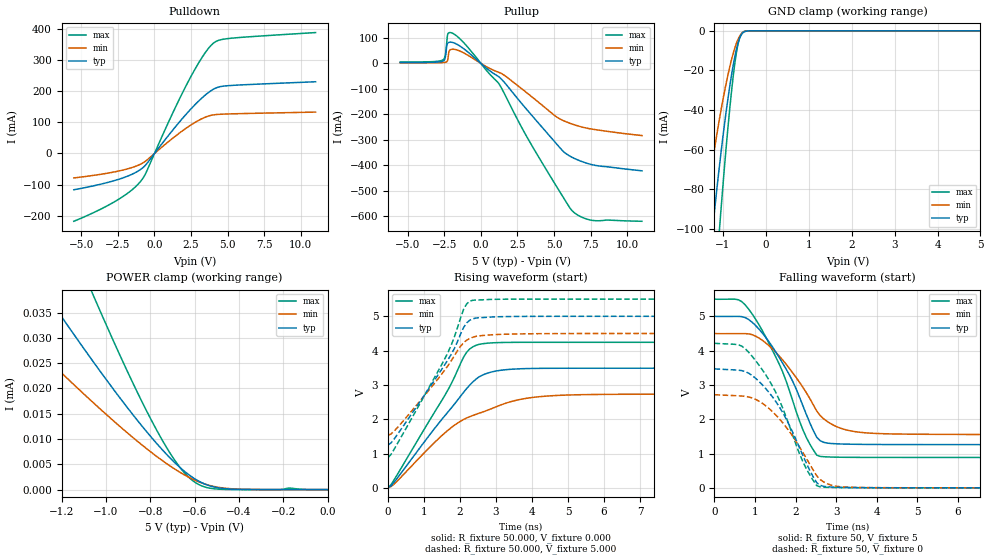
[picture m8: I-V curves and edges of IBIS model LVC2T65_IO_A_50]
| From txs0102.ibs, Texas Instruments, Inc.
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[Model]   LVC2T65_IO_A_50
Model_type  I/O
Vinl=0.15
Vinh=5.1
Enable   Active-High
Vref =   5
Rref =   1000000
Cref =   15p
Vmeas =   2.5
| variable   typ   min   max
C_comp   4.98pF   4.34pF   5.61pF
| C_pullup   5.82pF   4.29pF   6.44pF
| C_pulldown   5.22pF   5.04pF   5.82pF
| C_tri-state   4.98pF   4.34pF   5.61pF
[Temperature Range]   40   100   -40
| Ambient temperature   25   85   -40
[Voltage range]   5   4.5   5.5
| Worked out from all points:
|   slope of the pulldown table from 0 to 0.75 V, typ, clamps not added: 16.4 ohm
|   slope of the pullup table from 0 to 0.75 V, typ, clamps not added: 21.5 ohm
|   GND clamp passes 1 mA (typ) near -0.54 V on its own axis
|   rising waveform, R_fixture 50.000, V_fixture 0.000: 20-80 % time 1.54ns typ, 1.95ns min, 1.39ns max; typ from 0.006 V to 3.47 V
|   falling waveform, R_fixture 50, V_fixture 5: 20-80 % time 965ps typ, 1.04ns min, 960ps max; typ from 5 V to 1.26 V
|   rising waveform, R_fixture 50.000, V_fixture 5.000: 20-80 % time 1.37ns typ, 1.31ns min, 1.36ns max; typ from 1.25 V to 5 V
|   falling waveform, R_fixture 50, V_fixture 0: 20-80 % time 926ps typ, 951ps min, 930ps max; typ from 3.47 V to 0.006 V
[GND Clamp]
| LVC2T65_IO_A_50
|   Voltage   I(typ)   I(min)   I(max)
-5.5V     -1.326A    -1A        -1.717A
-1.455V   -147mA     -97.65mA   -214.4mA
-1.23V    -97.21mA   -63.81mA   -143mA
-1.085V   -68.32mA   -44.6mA    -100.4mA
-1.065V   -64.58mA   -42.12mA   -94.86mA
-900mV    -36.32mA   -23.63mA   -52.1mA
-815mV    -23.94mA   -15.61mA   -33.1mA
-740mV    -14.6mA    -9.631mA   -18.84mA
-685mV    -8.985mA   -6.069mA   -10.57mA
-630mV    -4.728mA   -3.343mA   -4.748mA
-515mV    -607.1uA   -516.6uA   -342.9uA
5V        589.8pA    504.4nA    134.3pA
[POWER Clamp]
| LVC2T65_IO_A_50
|   Voltage   I(typ)   I(min)   I(max)
-5.5V     360.2uA    239.1uA    590.4uA
-1.545V   56.8uA     37.99uA    90.83uA
-1.275V   38.94uA    26.19uA    61.14uA
-1.22V    35.41uA    23.86uA    55.27uA
-1.06V    25.42uA    17.28uA    38.66uA
-860mV    13.77uA    9.619uA    19.36uA
-775mV    9.301uA    6.68uA     12.04uA
-690mV    5.345uA    4.068uA    5.807uA
-615mV    2.578uA    2.192uA    1.98uA
-555mV    1.109uA    1.113uA    524.4nA
-460mV    171.6nA    258.4nA    30.67nA
0V        0A         0A         0A
[Pulldown]
| LVC2T65_IO_A_50
|   Voltage   I(typ)   I(min)   I(max)
-5.5V     -116.4mA   -78.48mA   -217.6mA
-2.54V    -84.37mA   -57.34mA   -149.8mA
-1.565V   -67.49mA   -45.7mA    -118.1mA
-900mV    -49.79mA   -33.28mA   -87.01mA
-580mV    -36.06mA   -23.83mA   -62.67mA
1.1V      66.05mA    43.19mA    114.4mA
2.34V     135mA      86.71mA    233.3mA
3.325V    181.5mA    113.4mA    313.3mA
4.045V    206.6mA    123.9mA    354.5mA
4.46V     214.1mA    125.7mA    364.1mA
5.2V      218.1mA    127mA      369.6mA
11V       230.1mA    132.8mA    388mA
[Pullup]
| LVC2T65_IO_A_50
|   Voltage   I(typ)   I(min)   I(max)
-5.5V     3.162mA    1.823mA    4.944mA
-2.61V    7.961mA    2.886mA    12.59mA
-2.425V   23.18mA    4mA        31.63mA
-2.24V    79.82mA    18.59mA    116.2mA
-2.135V   82.72mA    49.9mA     120.5mA
-1.785V   79.14mA    54.78mA    113.5mA
1.25V     -53.61mA   -35.9mA    -81.16mA
3.36V     -196.1mA   -125.6mA   -310mA
5.165V    -315.8mA   -210mA     -482.7mA
6.255V    -369.5mA   -238.7mA   -579.6mA
7.615V    -398mA     -258.5mA   -616.3mA
11V       -421.8mA   -283.5mA   -619.9mA
[Ramp]
| LVC2T65_IO_A_50
| variable   typ   min   max
dV/dt_r   2.17/1.55E-09   1.72/1.98E-09   2.63/1.40E-09
dV/dt_f   2.25/9.65E-10   1.78/1.04E-09   2.77/9.61E-10
R_load = 50
[Rising Waveform]
R_fixture = 50.000
V_fixture = 0.000
V_fixture_min = 0.000
V_fixture_max = 0.000
C_fixture = 0.000
L_fixture = 0.000
|  time   V(typ)   V(min)   V(max)
0s        6.039mV    5.318mV    6.534mV
168ps     168.5mV    116.3mV    239.8mV
1.596ns   2.128V     1.622V     2.732V
2.184ns   2.897V     2.04V      3.954V
2.352ns   3.086V     2.111V     4.109V
2.688ns   3.317V     2.235V     4.209V
3.528ns   3.465V     2.547V     4.242V
4.956ns   3.488V     2.707V     4.243V
8.316ns   3.489V     2.733V     4.242V
419.9ns   3.471V     2.719V     4.216V
[Falling Waveform]
| LVC2T65_IO_A_50
R_fixture =   50
C_fixture =   0
L_fixture =   0
V_fixture =   5
V_fixture_min = 4.5
V_fixture_max = 5.5
|   Time   V(typ)   V(min)   V(max)
0s        5V         4.5V       5.5V
588ps     4.998V     4.496V     5.481V
840ps     4.908V     4.488V     5.212V
1.764ns   3.466V     3.607V     3.119V
2.184ns   2.378V     2.921V     1.679V
2.436ns   1.669V     2.42V      1.106V
2.688ns   1.332V     2.016V     911.5mV
3.192ns   1.28V      1.71V      895.3mV
9.156ns   1.263V     1.553V     889.5mV
419.9ns   1.258V     1.541V     887.6mV
[Rising Waveform]
R_fixture = 50.000
V_fixture = 5.000
V_fixture_min = 4.500
V_fixture_max = 5.500
C_fixture = 0.000
L_fixture = 0.000
|  time   V(typ)   V(min)   V(max)
0s        1.253V     1.535V     884.1mV
336ps     1.675V     1.851V     1.436V
1.596ns   3.624V     3.464V     3.805V
1.764ns   3.91V      3.719V     4.186V
2.016ns   4.487V     4.131V     4.957V
2.1ns     4.676V     4.232V     5.205V
2.184ns   4.808V     4.304V     5.361V
2.436ns   4.948V     4.415V     5.475V
3.276ns   4.992V     4.479V     5.498V
419.9ns   5V         4.5V       5.5V
[Falling Waveform]
| LVC2T65_IO_A_50
R_fixture =   50
C_fixture =   0
L_fixture =   0
V_fixture =   0
V_fixture_min = 0
V_fixture_max = 0
|   Time   V(typ)   V(min)   V(max)
0s        3.47V      2.718V     4.215V
588ps     3.431V     2.685V     4.17V
840ps     3.345V     2.652V     3.955V
1.26ns    2.899V     2.396V     3.3V
1.596ns   2.365V     2.018V     2.565V
2.184ns   930.9mV    1.022V     749.7mV
2.52ns    152.2mV    353.2mV    69.06mV
2.772ns   37.68mV    127.2mV    20.95mV
3.192ns   15.96mV    30.02mV    11.14mV
419.9ns   5.773mV    4.795mV    6.514mV
